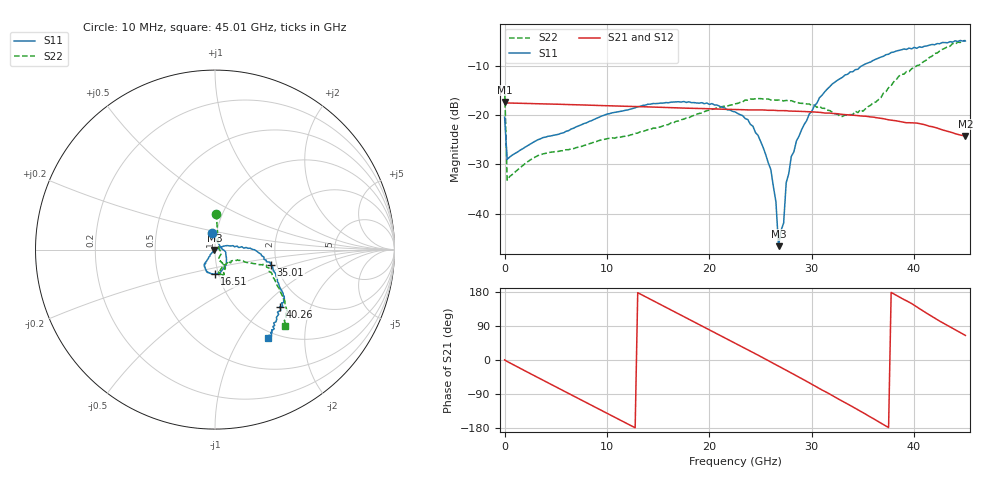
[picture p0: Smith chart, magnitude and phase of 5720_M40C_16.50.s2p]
! Device:  ADRF5720
! Description: 0.5dB LSB GaAs MMIC 6-bit Digital Attenuator
! Frequency:  0.000009 -  40 GHz
! Ports:
!	RF1	= Port 1
!	RF2	= Port 2
! Vdd:  3.3 Volt
! Vss:  -3.3 Volt
! Control:  0/3.3 Volt
! State:  16.50 dB attenuation
! Data:  The device was measured using G-S-G Probes on a matrix board.
!  Data was collected using an calibrated 4 port network analyzer.
!  The reference plane for this measurement is at the launchers.
! Note:  Analog Devices supplies this data as a sample of measured data
!  for this product.  Your particular data for this product may vary.
!  Data was taken at -40 degrees C.
!  Analog Devices reserves the right to change this data at anytime.
# GHZ S DB R 45.0
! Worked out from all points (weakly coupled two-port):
!   181 points, 10 MHz to 45.01 GHz, reference 45 ohm
!   highest |S21| = -17.30 dB at 10 MHz (marker M1); lowest = -24.2 dB at 45.01 GHz (marker M2)
!   lowest |S11| = -46.6 dB at 26.76 GHz (marker M3), VSWR 1.01, Z = 44.7 - j0.243 ohm
!   |S11| at or under -10 dB: start of sweep to 34.83 GHz
!   |S22| runs from -33.2 to -4.8 dB; largest |S21 - S12| = 0.00049
!   S11 on the Smith chart (normalised r, x): 10 MHz: 0.95, +0.18; 16.51 GHz: 0.96, -0.27; 35.01 GHz: 1.86, -0.36; 40.26 GHz: 1.51, -1.25; 45.01 GHz: 0.91, -1.32
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0.01  -20.36 101.5  -17.30 0.2  -17.32 0.2  -14.01 88.0
0.26  -28.96 14.7  -17.48 -3.9  -17.49 -3.9  -33.20 21.4
3.26  -24.97 -9.4  -17.64 -46.3  -17.66 -46.4  -28.19 -29.2
7.76  -21.67 -39.2  -17.89 -109.2  -17.91 -109.2  -26.14 -61.5
11.76  -19.00 -62.5  -18.15 -165.0  -18.17 -165.0  -24.26 -67.2
15.26  -17.50 -83.3  -18.36 146.0  -18.38 145.9  -22.32 -63.5
16.51  -17.29 -91.0  -18.46 128.5  -18.48 128.5  -21.55 -61.5
20.26  -17.60 -110.5  -18.68 76.0  -18.70 75.9  -18.78 -61.4
22.76  -19.60 -125.4  -18.83 41.0  -18.85 40.9  -17.57 -67.9
24.26  -22.21 -126.5  -18.90 20.0  -18.92 19.9  -16.71 -70.3
26.01  -31.05 -132.9  -18.96 -5.2  -18.99 -5.4  -16.87 -74.5
26.51  -37.65 -125.1  -19.01 -12.7  -19.03 -12.9  -16.92 -76.7
26.76  -46.64 -144.2  -19.04 -16.2  -19.06 -16.4  -16.87 -75.3
27.26  -41.93 36.3  -19.05 -23.4  -19.07 -23.6  -17.06 -76.5
27.51  -33.72 14.0  -19.05 -27.1  -19.07 -27.2  -16.95 -77.9
28.01  -28.35 19.5  -19.13 -34.3  -19.15 -34.5  -17.01 -79.2
30.26  -18.06 8.9  -19.32 -67.7  -19.35 -67.8  -17.91 -78.8
32.76  -12.55 -2.7  -19.75 -105.2  -19.78 -105.3  -20.20 -64.4
35.01  -9.79 -15.6  -20.16 -138.9  -20.18 -139.0  -19.17 -34.9
37.76  -7.20 -31.6  -20.99 178.3  -21.01 178.1  -13.98 -21.2
40.26  -6.35 -41.4  -21.57 140.2  -21.58 140.0  -9.88 -18.9
45.01  -4.86 -59.2  -24.21 64.9  -24.24 64.7  -4.77 -47.2
